(* Logix 5000 AddOnInstructionDefinition export Banner_LE_PD_v4; software revision 33.00 *)

TYPE Banner_LE_PDI_v4 :   // UDT that records the converted prcoess data.
STRUCT
   Channel_1_Output_State : SINT;   // 0 = Inactive, 1 = Active
   Channel_2_Output_State : SINT;   // 0 = Inactive, 1 = Active
   Sensor_Stability : SINT;   // 0 = No target or Marginal signal, 1 = Stable signal
   Measurement_Value : REAL;   // Distance from sensor face in mm's.
   PDI_DT : SINT[4];   // Data Transfer array for Process Data Input.
END_STRUCT
END_TYPE

ADD_ON_INSTRUCTION Banner_LE_PD_v4   (* revision 4.0, vendor Banner Engineering *)
// Takes the raw SINT information and converts that data into actual information.
VAR_IN_OUT
   Process_Data : Banner_LE_PDI_v4; {required}
END_VAR
VAR_INPUT
   Byte_Swap : BOOL; {required}
END_VAR
VAR
   Temp_Measurement : DINT; {access None}
   Temp_Byte_Array : SINT[4]; {access None}
END_VAR

ROUTINE Logic   (* ladder *)
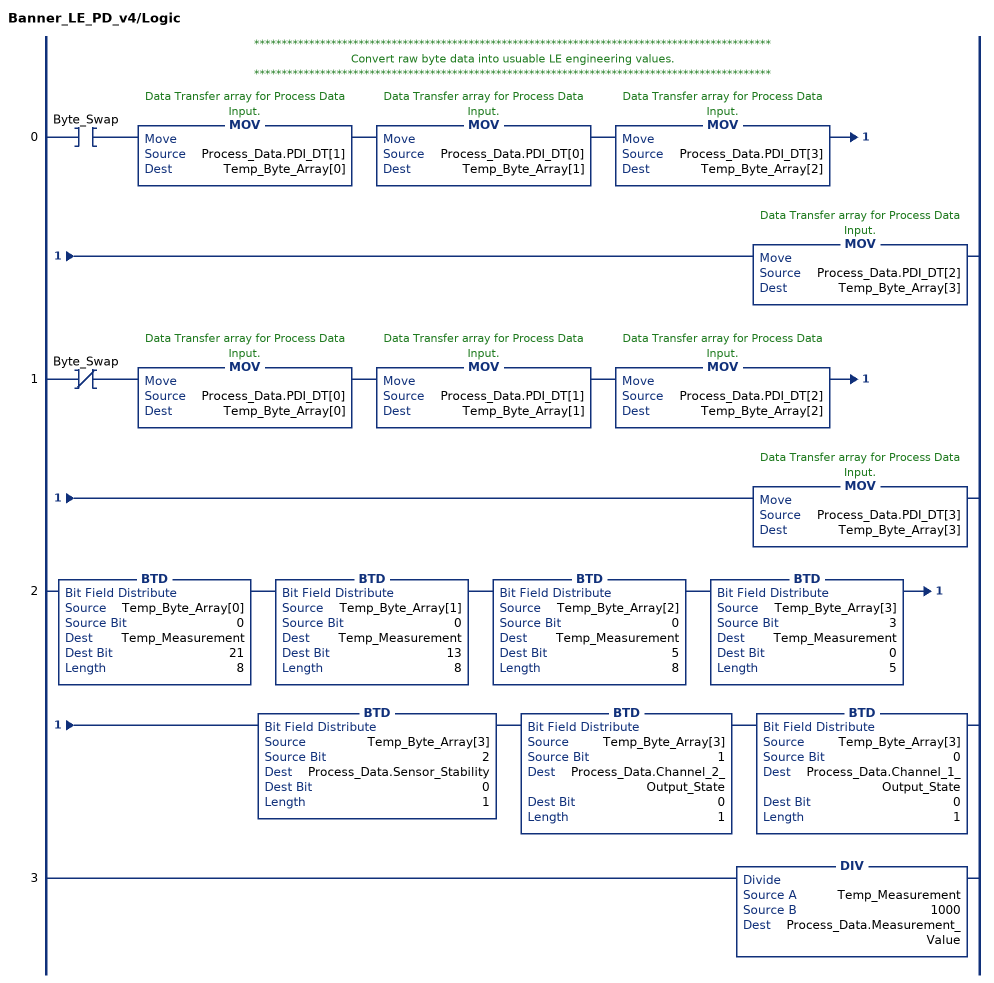
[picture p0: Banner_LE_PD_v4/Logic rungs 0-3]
   // **********************************************************************************************
   // Convert raw byte data into usuable LE engineering values.
   // **********************************************************************************************
   0: XIC(Byte_Swap)MOV(Process_Data.PDI_DT[1],Temp_Byte_Array[0])MOV(Process_Data.PDI_DT[0],Temp_Byte_Array[1])MOV(Process_Data.PDI_DT[3],Temp_Byte_Array[2])MOV(Process_Data.PDI_DT[2],Temp_Byte_Array[3]);
   1: XIO(Byte_Swap)MOV(Process_Data.PDI_DT[0],Temp_Byte_Array[0])MOV(Process_Data.PDI_DT[1],Temp_Byte_Array[1])MOV(Process_Data.PDI_DT[2],Temp_Byte_Array[2])MOV(Process_Data.PDI_DT[3],Temp_Byte_Array[3]);
   2: BTD(Temp_Byte_Array[0],0,Temp_Measurement,21,8)BTD(Temp_Byte_Array[1],0,Temp_Measurement,13,8)BTD(Temp_Byte_Array[2],0,Temp_Measurement,5,8)BTD(Temp_Byte_Array[3],3,Temp_Measurement,0,5)BTD(Temp_Byte_Array[3],2,Process_Data.Sensor_Stability,0,1)BTD(Temp_Byte_Array[3],1,Process_Data.Channel_2_Output_State,0,1)BTD(Temp_Byte_Array[3],0,Process_Data.Channel_1_Output_State,0,1);
   3: DIV(Temp_Measurement,1000,Process_Data.Measurement_Value);
END_ROUTINE
END_ADD_ON_INSTRUCTION
